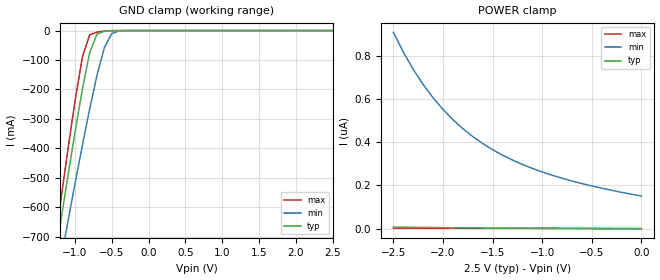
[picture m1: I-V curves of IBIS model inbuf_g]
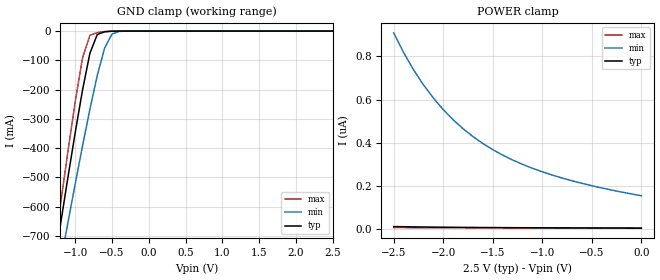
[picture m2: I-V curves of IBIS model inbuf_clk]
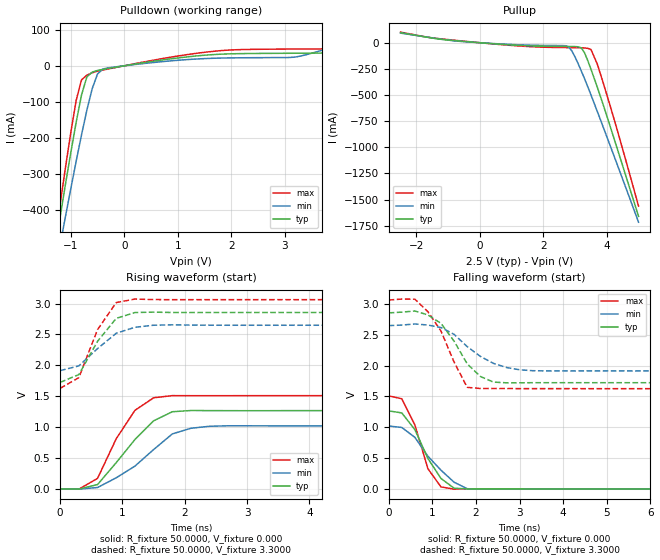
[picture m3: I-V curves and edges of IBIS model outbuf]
| IBIS file 5v2310z_tssop_2p5.ibs created by s2ibis2 version 1.2
| North Carolina State University Electronics Research Laboratory  1995
[IBIS ver]   2.1
[File name]   5v2310z.ibs
[File Rev]   0.4
[Date]   02/26/2004 jbp
[Source]   Integrated Device Technology, Inc.
[Notes]   1.Temperatures: typ=25C, min=150C, max=-40C 2.RRmp rates based
   on 500 ohm load and 25pF.
[Disclaimer] Integrated Device Technology, Inc. ("IDT") hereby grants the
   user of this IBIS model a non-exclusive, nontransferable
   license to use this IBIS model under the following terms. The
   user is granted this license only to use the IBIS model and is
   not granted rights to sell, copy (except as needed to run the
   IBIS model), rent, lease or sub-license the IBIS model in
   whole or in part, or in modified form to anyone. The User may
   modify the IBIS model to suit its specific applications, but
   rights to derivative works and such modifications shall belong
   to IDT. This IBIS model is provided on an AS IS" basis and IDT
   makes absolutely no warranty with respect to the information
   contained herein. IDT DISCLAIMS AND CUSTOMER WAIVES ALL
   WARRANTIES, EXPRESS AND IMPLIED, INCLUDING WARRANTIES OF
   MERCHANTABILITY AND FITNESS FOR A PARTICULAR PURPOSE. THE
   ENTIRE RISK AS TO QUALITY AND PERFORMANCE IS WITH THE USER
   ACCORDINGLY, IN NO EVENT SHALL IDT BE LIABLE FOR ANY DIRECT OR
   INDIRECT DAMAGES, WHETHER IN CONTRACT OR TORT, INCLUDING ANY
   LOST PROFITS OR OTHER INCIDENTAL, CONSEQUENTIAL, EXEMPLARY, OR
   PUNITIVE DAMAGES ARISING OUT OF THE USE OR APPLICATION OF THE
   IBIS model. Further, IDT reserves the right to make changes
   without notice to any product herein to improve reliability,
   function, or design. IDT does not convey any license under
   patent rights or any other intellectual property rights,
   including those of third parties. IDT is not obligated to
   provide maintenance or support for the licensed IBIS model.
[Copyright]   Copyright 1997, Integrated Device Technology, Inc. all rights
   reserved
|   Component idt5v2310z
[Component]   idt5v2310z
[Manufacturer]   Integrated Device Technology, Inc.
[Package]
| variable   typ   min   max
R_pkg   91.60m   81.80m   101.4m
L_pkg   3.14nH   2.64nH   3.65nH
C_pkg   0.390pF   0.314pf   0.462pF
[Pin]  signal_name   model_name   R_pin   L_pin   C_pin
1   GND   GND
2   VDD   POWER
3   Y10   outbuf
4   Y11   outbuf
5   Y12   outbuf
6   GND   GND
7   GND   GND
8   Y13   outbuf
9   Y14   outbuf
10   VDD   POWER
11   G1   inbuf_g
12   Y24   outbuf
13   G2   inbuf_g
14   VDD   POWER
15   VDD   POWER
16   Y23   outbuf
17   Y22   outbuf
18   GND   GND
19   GND   GND
20   Y21   outbuf
21   Y20   outbuf
22   VDD   POWER
23   VDD   POWER
24   CLK   inbuf_clk
| Models and submodels in the file (3): inbuf_g (Input), inbuf_clk (Input), outbuf (Output)
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|   Model inbuf_g
[Model]   inbuf_g
Model_type   Input
Polarity   Non-Inverting
Vinl =   0.7000V
Vinh =   1.7000V
C_comp   3.0000pF   NA   NA
[Temperature Range]   25.0000   0.1500k   -40.0000
[Voltage Range]   2.5000V   2.3000V   2.7000V
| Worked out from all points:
|   GND clamp passes 1 mA (typ) near -0.52 V on its own axis
[GND_clamp]
| voltage   I(typ)   I(min)   I(max)
-2.5V     -2.824A    -2.624A    -3.04A
-1.3V     -823mA     -929.4mA   -775.2mA
-1.2V     -661.4mA   -792.1mA   -592.7mA
-1.1V     -502.3mA   -656.3mA   -413.9mA
-1V       -347.6mA   -522.7mA   -242.5mA
-900mV    -201.2mA   -392.2mA   -91.4mA
-800mV    -75.82mA   -267mA     -14.55mA
-700mV    -11.63mA   -151.7mA   -5.267mA
-600mV    -2.491mA   -58.09mA   -1.497mA
-500mV    -519.6uA   -10.16mA   -175.5uA
-400mV    -56.6uA    -1.033mA   -10.24uA
2.5V      370pA      168nA      -198.5pA
[POWER_clamp]
| voltage   I(typ)   I(min)   I(max)
-2.5V     7.545nA    907.1nA    2.543nA
-2.4V     6.793nA    816nA      2.437nA
-2.3V     6.132nA    736.1nA    2.331nA
-2.2V     5.55nA     666.1nA    2.227nA
-2.1V     5.036nA    604.7nA    2.123nA
-1.9V     4.174nA    503.7nA    1.917nA
-1.8V     3.81nA     462.2nA    1.815nA
-1.6V     3.189nA    393.5nA    1.611nA
-1.3V     2.447nA    317.1nA    1.307nA
-1V       1.855nA    262.1nA    1.005nA
-600mV    1.2nA      208.5nA    603.2pA
0V        370pA      150.9nA    1.777pA
|   Model inbuf_clk
[Model]   inbuf_clk
Model_type   Input
Polarity   Non-Inverting
Vinl =   0.7000V
Vinh =   1.7000V
C_comp   3.0000pF   NA   NA
[Temperature Range]   25.0000   0.1500k   -40.0000
[Voltage Range]   2.5000V   2.3000V   2.7000V
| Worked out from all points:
|   GND clamp passes 1 mA (typ) near -0.52 V on its own axis
[GND_clamp]
| voltage   I(typ)   I(min)   I(max)
-2.5V     -2.824A    -2.624A    -3.04A
-1.3V     -823mA     -929.4mA   -775.2mA
-1.2V     -661.4mA   -792.1mA   -592.7mA
-1.1V     -502.3mA   -656.3mA   -413.9mA
-1V       -347.6mA   -522.7mA   -242.5mA
-900mV    -201.2mA   -392.2mA   -91.4mA
-800mV    -75.82mA   -267mA     -14.55mA
-700mV    -11.63mA   -151.7mA   -5.267mA
-600mV    -2.491mA   -58.09mA   -1.497mA
-500mV    -519.6uA   -10.16mA   -175.5uA
-400mV    -56.6uA    -1.033mA   -10.24uA
2.5V      2.87nA     170.3nA    2.501nA
[POWER_clamp]
| voltage   I(typ)   I(min)   I(max)
-2.5V     10.05nA    909.4nA    5.243nA
-2.4V     9.293nA    818.3nA    5.137nA
-2.3V     8.632nA    738.4nA    5.031nA
-2.2V     8.05nA     668.4nA    4.927nA
-2.1V     7.536nA    607nA      4.823nA
-1.9V     6.674nA    506nA      4.617nA
-1.8V     6.31nA     464.5nA    4.515nA
-1.6V     5.689nA    395.8nA    4.311nA
-1.3V     4.947nA    319.4nA    4.007nA
-1V       4.355nA    264.4nA    3.705nA
-600mV    3.7nA      210.8nA    3.303nA
0V        2.87nA     153.2nA    2.702nA
|   Model outbuf
[Model]   outbuf
Model_type   Output
Polarity   Non-Inverting
Vmeas =   1.2500V
Cref =  25.0000pF
Rref =   0.5000k
C_comp   3.0000pF   NA   NA
[Temperature Range]   25.0000   0.1500k   -40.0000
[Voltage Range]   2.5000V   2.3000V   2.7000V
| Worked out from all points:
|   slope of the pulldown table from 0 to 0.375 V, typ, clamps not added: 42.2 ohm
|   slope of the pullup table from 0 to 0.375 V, typ, clamps not added: 42.8 ohm
|   rising waveform, R_fixture 50.0000, V_fixture 0.000: 20-80 % time 657ps typ, 773ps min, 496ps max; typ from 0 V to 1.27 V
|   rising waveform, R_fixture 50.0000, V_fixture 3.3000: 20-80 % time 439ps typ, 504ps min, 392ps max; typ from 1.72 V to 2.86 V
|   falling waveform, R_fixture 50.0000, V_fixture 0.000: 20-80 % time 578ps typ, 732ps min, 443ps max; typ from 1.27 V to 0 V
|   falling waveform, R_fixture 50.0000, V_fixture 3.3000: 20-80 % time 659ps typ, 829ps min, 611ps max; typ from 2.86 V to 1.72 V
[Pulldown]
| voltage   I(typ)   I(min)   I(max)
-2.5V     -1.657A    -1.549A    -1.777A
-1.3V     -509.5mA   -574.3mA   -484.7mA
-1.1V     -327.5mA   -416.9mA   -281.3mA
-900mV    -156.1mA   -264.2mA   -95.56mA
-800mV    -80.79mA   -191.3mA   -38.93mA
-700mV    -30.75mA   -122.9mA   -26.02mA
-500mV    -12.88mA   -22.66mA   -15mA
-400mV    -9.924mA   -8.915mA   -11.88mA
1.6V      30.36mA    20.52mA    39.03mA
3.2V      34.78mA    24.17mA    46.42mA
4.3V      60.41mA    69.8mA     51.29mA
5V        97.52mA    102mA      90.99mA
[Pullup]
| voltage   I(typ)   I(min)   I(max)
-2.5V     96.57mA    91.98mA    101.7mA
-600mV    15.14mA    12.35mA    17.81mA
1.3V      -26.32mA   -20.63mA   -32.38mA
2.7V      -35.48mA   -28.75mA   -46.51mA
2.8V      -35.71mA   -40.76mA   -46.85mA
2.9V      -35.98mA   -79.47mA   -47.18mA
3.2V      -50.06mA   -272.5mA   -48.25mA
3.3V      -97.84mA   -345.3mA   -49.91mA
3.5V      -252.4mA   -498.6mA   -64.25mA
3.7V      -424.9mA   -656.9mA   -204.1mA
4.3V      -985.1mA   -1.142A    -804.4mA
5V        -1.66A     -1.716A    -1.562A
[Ramp]
| variable   typ   min   max
dV/dt_r   1.3836/0.5014n   1.2480/0.6774n   1.5138/0.3902n
dV/dt_f   1.3855/0.5823n   1.2388/0.7547n   1.5172/0.4708n
R_load = 0.5000k
[Rising Waveform]
R_fixture = 50.0000
V_fixture = 0.000
| time   V(typ)   V(min)   V(max)
0s        -83.75uV   -43.38uV   -133.1uV
300ps     -5.315mV   -4.394mV   -5.63mV
600ps     68.93mV    21.07mV    168.7mV
900ps     424.2mV    178.7mV    811.5mV
1.2ns     798.3mV    367.7mV    1.271V
1.5ns     1.101V     636.3mV    1.474V
1.8ns     1.248V     889.4mV    1.51V
2.1ns     1.268V     981.1mV    1.508V
2.7ns     1.266V     1.021V     1.508V
15ns      1.266V     1.02V      1.509V
[Rising Waveform]
R_fixture = 50.0000
V_fixture = 3.3000
V_fixture_min = 3.0000
V_fixture_max = 3.6000
| time   V(typ)   V(min)   V(max)
0s        1.724V     1.914V     1.627V
300ps     1.851V     1.991V     1.801V
600ps     2.389V     2.271V     2.578V
900ps     2.76V      2.519V     3.017V
1.2ns     2.855V     2.616V     3.073V
1.5ns     2.861V     2.649V     3.065V
1.8ns     2.856V     2.656V     3.063V
2.7ns     2.856V     2.649V     3.064V
15ns      2.856V     2.649V     3.064V
[Falling Waveform]
R_fixture = 50.0000
V_fixture = 0.000
| time   V(typ)   V(min)   V(max)
0s        1.266V     1.02V      1.509V
300ps     1.232V     996.8mV    1.462V
600ps     962.2mV    836.4mV    1.038V
900ps     492mV      529.6mV    325.3mV
1.2ns     168.6mV    302.3mV    31.81mV
1.5ns     10.75mV    107.8mV    -4.591mV
1.8ns     -291.5uV   2.83mV     1.927mV
2.1ns     1.631mV    -4.111mV   1.292mV
2.7ns     740.4uV    1.009mV    495uV
15ns      0V         1.436uV    0V
[Falling Waveform]
R_fixture = 50.0000
V_fixture = 3.3000
V_fixture_min = 3.0000
V_fixture_max = 3.6000
| time   V(typ)   V(min)   V(max)
0s        2.856V     2.649V     3.064V
600ps     2.886V     2.676V     3.079V
900ps     2.822V     2.659V     2.874V
1.2ns     2.685V     2.618V     2.56V
1.5ns     2.396V     2.507V     2.056V
1.8ns     2.029V     2.308V     1.647V
2.1ns     1.825V     2.151V     1.629V
2.4ns     1.733V     2.037V     1.628V
3.3ns     1.723V     1.917V     1.627V
15ns      1.723V     1.914V     1.626V
